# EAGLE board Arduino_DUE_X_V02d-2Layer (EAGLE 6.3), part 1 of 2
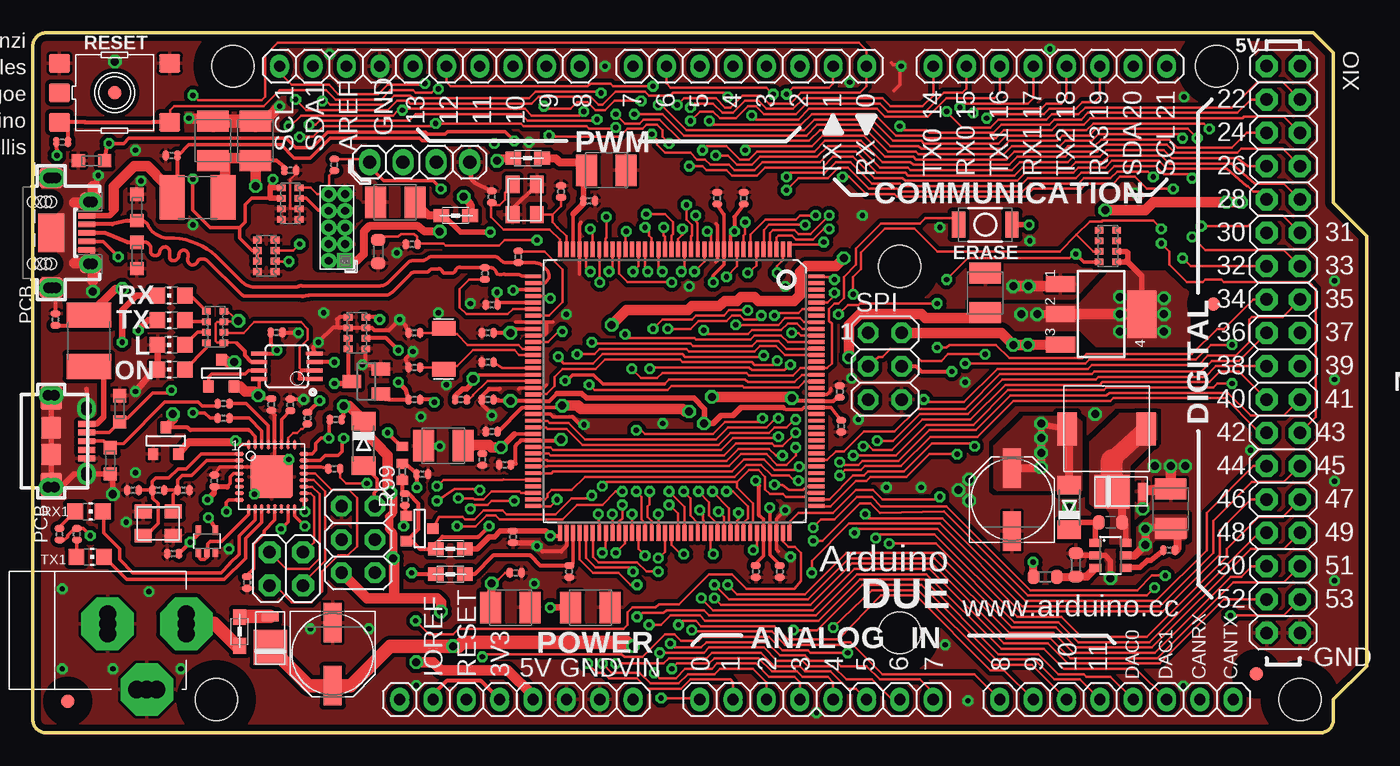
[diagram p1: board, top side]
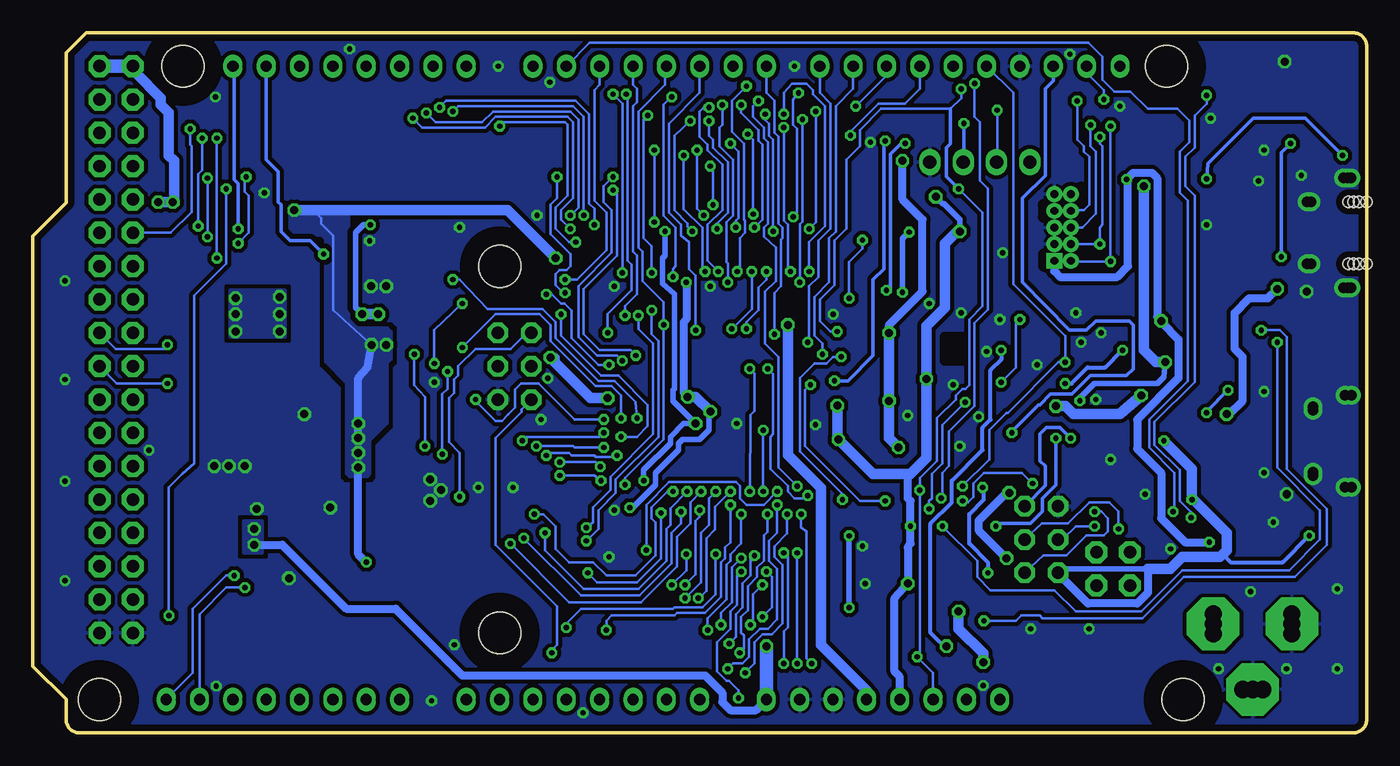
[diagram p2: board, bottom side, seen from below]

Size 101.6 x 53.34 mm. Coordinates in mm from the lower left corner, seen from the top.
Outline: 97.54,53.34 99.06,51.82 99.06,40.39 101.6,37.85 101.6,5.08 99.06,2.54 99.06,1 arc-90 98.06,0 1,0 arc-90 0,1 0,52.34 arc-90 1,53.34 97.54,53.34
Copper layers (1*16): Top 0.035mm / dielectric 1.6mm / Bottom 0.035mm
Design rules "default *": minimum track width 8mil, minimum drill 16mil, track to track 8mil, track to pad 8mil, pad to pad 8mil, via to via 8mil, smd to smd 6mil, copper to edge 20mil, drill to drill 12mil, minimum pad ring 12mil, minimum via ring 8mil, stop-mask expansion 2mil, vias tented up to drill 25mil, thermal gap 8mil
Net classes: 0 default: width 0.203 mm, drill 0.406 mm, clearance 0.203 mm; 1 USB: width 0.203 mm, drill 0.406 mm, clearance 0.203 mm; 2 gnd: width 0.203 mm, drill 0.406 mm, clearance 0.203 mm; 3 usbvcc: width 0.203 mm, drill 0.406 mm, clearance 0.203 mm; 4 USBpair: width 0.254 mm, drill 0.406 mm, clearance 0.61 mm
Holes 3.2 mm at 96.52,2.54 15.24,50.8 90.17,50.8 13.97,2.54 66.04,35.56 66.04,7.62
tRestrict: area 63.5,5.1 to 68.6,10.2; area 12.7,48.3 to 17.8,53.3; area 63.5,33 to 68.6,38.1; area 87.6,48.3 to 92.7,53.3; area 94,0 to 99.1,5.1; area 11.4,0 to 16.5,5.1; 5 lines
bRestrict: area 63.5,5.1 to 68.6,10.2; area 12.7,48.3 to 17.8,53.3; area 63.5,33 to 68.6,38.1; area 87.6,48.3 to 92.7,53.3; area 94,0 to 99.1,5.1; area 11.4,0 to 16.5,5.1; 5 lines

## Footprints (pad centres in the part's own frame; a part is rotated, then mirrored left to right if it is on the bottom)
1X08 = drill 0.85 pad 1.422 long: 1 -8.89,0; 2 -6.35,0; 3 -3.81,0; 4 -1.27,0; 5 1.27,0; 6 3.81,0; 7 6.35,0; 8 8.89,0
J0402 = smd 0.7 x 0.9: 1 -0.65,0; 2 0.65,0; 3 1.95,0
SMC_B = smd 1.6 x 2.4: + -1.5,0; - 1.5,0
C0402 = smd 0.508 x 0.762: 1 -0.445,0; 2 0.445,0
C0603-ROUND = smd 0.898 x 1.1: 1 -0.889,0; 2 0.889,0
MINIMELF = smd 1.4 x 1.8: A 1.7,0; C -1.7,0
DO220AAL = smd 2.667 x 2.54: P$1 -0.7,0 | smd 0.762 x 1.27: P$2 1.65,0
1X04 = drill 1.016 long: 1 -3.81,0; 2 -1.27,0; 3 1.27,0; 4 3.81,0
SMD_157SW = smd 1.016 x 1.981: 1 -2.032,0; 2 2.032,0
L1812 = smd 1.9 x 3.4: 1 -1.95,0; 2 1.95,0
FIDUCIA-MOUNT = smd 1.016 x 1.016: P$1 0,0
MSOP08 = smd 0.3 x 1.2: 1 -0.976,-2.113; 2 -0.326,-2.113; 3 0.324,-2.113; 4 0.974,-2.113; 5 0.974,2.112; 6 0.324,2.112; 7 -0.326,2.112; 8 -0.976,2.112
SOT23-6 = smd 0.6 x 0.9: 1 -0.95,-1.15; 2 0,-1.15; 3 0.95,-1.15; 4 0.95,1.15; 5 0,1.15; 6 -0.95,1.15
SOT223 = smd 1.219 x 2.235: 1 -2.311,-3.099; 2 0,-3.099; 3 2.311,-3.099 | smd 3.6 x 2.2: 4 0,3.099
MLF32 = smd 0.7 x 0.28: 1 -2.45,1.75; 2 -2.45,1.25; 3 -2.45,0.75; 4 -2.45,0.25; 5 -2.45,-0.25; 6 -2.45,-0.75; 7 -2.45,-1.25; 8 -2.45,-1.75; 17 2.45,-1.75; 18 2.45,-1.25; 19 2.45,-0.75; 20 2.45,-0.25; 21 2.45,0.25; 22 2.45,0.75; 23 2.45,1.25; 24 2.45,1.75 | smd 0.28 x 0.7: 9 -1.75,-2.45; 10 -1.25,-2.45; 11 -0.75,-2.45; 12 -0.25,-2.45; 13 0.25,-2.45; 14 0.75,-2.45; 15 1.25,-2.45; 16 1.75,-2.45; 25 1.75,2.45; 26 1.25,2.45; 27 0.75,2.45; 28 0.25,2.45; 29 -0.25,2.45; 30 -0.75,2.45; 31 -1.25,2.45; 32 -1.75,2.45 | smd 3.254 x 3.254: 33 0,0
SC70-5 = smd 0.4 x 0.7: 1 -0.65,-0.85; 2 0,-0.85; 3 0.65,-0.85; 4 0.65,0.85; 5 -0.65,0.85
2X03 = drill 0.95 pad 1.55 octagon: 1 -2.54,-1.27; 2 -2.54,1.27; 3 0,-1.27; 4 0,1.27; 5 2.54,-1.27; 6 2.54,1.27
CON2_USB_MICRO_B_AT = smd 0.406 x 1.346: P1 -1.321,2.692; P2 -0.66,2.692; P3 0,2.692; P4 0.66,2.692; P5 1.321,2.692 | drill 0.8 pad 1.27: P$1 -2.616,2.692 | drill 0.8 pad 1.245: P$2 -2.362,2.692; P$7 2.362,2.692; P$8 2.616,2.692 | drill 0.8 pad 1.143: P$3 -3.505,-0.254; P$4 -3.505,0.254; P$5 3.505,0.254; P$6 3.505,-0.254 | smd 1.778 x 1.651: S1 -3.302,0; S2 3.302,0 | smd 1.524 x 1.27: S3 -2.489,2.692; S4 2.489,2.692 | smd 1.626 x 1.524: S5 -1.016,0; S6 1.016,0
2X02 = drill 0.95 pad 1.676 octagon: 1 -1.27,-1.27; 2 -1.27,1.27; 3 1.27,-1.27; 4 1.27,1.27
R0402 = smd 0.508 x 0.762: 1 -0.445,0; 2 0.445,0
PINHEAD_2X05_127 = drill 0.6 pad 1.016 square: 1 -0.635,2.54 | drill 0.6 pad 1.016: 2 0.635,2.54; 3 -0.635,1.27; 4 0.635,1.27; 5 -0.635,0; 6 0.635,0; 7 -0.635,-1.27; 8 0.635,-1.27; 9 -0.635,-2.54; 10 0.635,-2.54
CHIP-LED0805 = smd 1.2 x 1.2: A 0,-1.05; C 0,1.05
0805 = smd 1.2 x 1: 1 -1.1,0; 2 1.1,0
SRR0604 = smd 1.5 x 2.5: P$1 3,0; P$2 -3,0
PANASONIC_D = smd 3 x 1.4: + 2.4,0; - -2.4,0
1X10 = drill 0.85 pad 1.422 long: 1 -11.43,0; 2 -8.89,0; 3 -6.35,0; 4 -3.81,0; 5 -1.27,0; 6 1.27,0; 7 3.81,0; 8 6.35,0; 9 8.89,0; 10 11.43,0
SOT23 = smd 1 x 1.4: 1 -0.95,-1.1; 2 0.95,-1.1; 3 0,1.1
R0603-ROUND = smd 0.898 x 1.1: 1 -0.889,0; 2 0.889,0
TS42 = smd 1.6 x 1.4: 1 -4.2,2.25; 2 4.2,2.25; 3 -4.2,-2.25; 4 4.2,-2.25; 5 -4.2,0
CAT16 = smd 0.5 x 0.65: 1 -1.2,-0.675; 2 -0.4,-0.675; 3 0.4,-0.675; 4 1.2,-0.675; 5 1.2,0.675; 6 0.4,0.675; 7 -0.4,0.675; 8 -1.2,0.675
CAY16 = smd 0.5 x 0.65: 1 -1.2,-0.675; 2 -0.4,-0.675; 3 0.4,-0.675; 4 1.2,-0.675; 5 1.2,0.675; 6 0.4,0.675; 7 -0.4,0.675; 8 -1.2,0.675
SOT-23 = smd 0.787 x 0.889: 1 0.025,-1.016; 2 -0.94,1.016; 3 0.991,1.016
LQFP144 = smd 0.3 x 1.2: 1 -8.75,-10.8; 2 -8.25,-10.8; 3 -7.75,-10.8; 4 -7.25,-10.8; 5 -6.75,-10.8; 6 -6.25,-10.8; 7 -5.75,-10.8; 8 -5.25,-10.8; 9 -4.75,-10.8; 10 -4.25,-10.8; 11 -3.75,-10.8; 12 -3.25,-10.8; 13 -2.75,-10.8; 14 -2.25,-10.8; 15 -1.75,-10.8; 16 -1.25,-10.8; 17 -0.75,-10.8; 18 -0.25,-10.8; 19 0.25,-10.8; 20 0.75,-10.8; 21 1.25,-10.8; 22 1.75,-10.8; 23 2.25,-10.8; 24 2.75,-10.8; 25 3.25,-10.8; 26 3.75,-10.8; 27 4.25,-10.8; 28 4.75,-10.8; 29 5.25,-10.8; 30 5.75,-10.8; 31 6.25,-10.8; 32 6.75,-10.8; 33 7.25,-10.8; 34 7.75,-10.8; 35 8.25,-10.8; 36 8.75,-10.8; 73 8.75,10.8; 74 8.25,10.8; 75 7.75,10.8; 76 7.25,10.8; 77 6.75,10.8; 78 6.25,10.8; 79 5.75,10.8; 80 5.25,10.8; 81 4.75,10.8; 82 4.25,10.8; 83 3.75,10.8; 84 3.25,10.8; 85 2.75,10.8; 86 2.25,10.8; 87 1.75,10.8; 88 1.25,10.8; 89 0.75,10.8; 90 0.25,10.8; 91 -0.25,10.8; 92 -0.75,10.8; 93 -1.25,10.8; 94 -1.75,10.8; 95 -2.25,10.8; 96 -2.75,10.8; 97 -3.25,10.8; 98 -3.75,10.8; 99 -4.25,10.8; 100 -4.75,10.8; 101 -5.25,10.8; 102 -5.75,10.8; 103 -6.25,10.8; 104 -6.75,10.8; 105 -7.25,10.8; 106 -7.75,10.8; 107 -8.25,10.8; 108 -8.75,10.8 | smd 1.2 x 0.3: 37 10.8,-8.75; 38 10.8,-8.25; 39 10.8,-7.75; 40 10.8,-7.25; 41 10.8,-6.75; 42 10.8,-6.25; 43 10.8,-5.75; 44 10.8,-5.25; 45 10.8,-4.75; 46 10.8,-4.25; 47 10.8,-3.75; 48 10.8,-3.25; 49 10.8,-2.75; 50 10.8,-2.25; 51 10.8,-1.75; 52 10.8,-1.25; 53 10.8,-0.75; 54 10.8,-0.25; 55 10.8,0.25; 56 10.8,0.75; 57 10.8,1.25; 58 10.8,1.75; 59 10.8,2.25; 60 10.8,2.75; 61 10.8,3.25; 62 10.8,3.75; 63 10.8,4.25; 64 10.8,4.75; 65 10.8,5.25; 66 10.8,5.75; 67 10.8,6.25; 68 10.8,6.75; 69 10.8,7.25; 70 10.8,7.75; 71 10.8,8.25; 72 10.8,8.75; 109 -10.8,8.75; 110 -10.8,8.25; 111 -10.8,7.75; 112 -10.8,7.25; 113 -10.8,6.75; 114 -10.8,6.25; 115 -10.8,5.75; 116 -10.8,5.25; 117 -10.8,4.75; 118 -10.8,4.25; 119 -10.8,3.75; 120 -10.8,3.25; 121 -10.8,2.75; 122 -10.8,2.25; 123 -10.8,1.75; 124 -10.8,1.25; 125 -10.8,0.75; 126 -10.8,0.25; 127 -10.8,-0.25; 128 -10.8,-0.75; 129 -10.8,-1.25; 130 -10.8,-1.75; 131 -10.8,-2.25; 132 -10.8,-2.75; 133 -10.8,-3.25; 134 -10.8,-3.75; 135 -10.8,-4.25; 136 -10.8,-4.75; 137 -10.8,-5.25; 138 -10.8,-5.75; 139 -10.8,-6.25; 140 -10.8,-6.75; 141 -10.8,-7.25; 142 -10.8,-7.75; 143 -10.8,-8.25; 144 -10.8,-8.75
MCR-AB1-S-RA-SMT = smd 0.4 x 1.35: 1 -1.3,2.7; 2 -0.65,2.7; 3 0,2.7; 4 0.65,2.7; 5 1.3,2.7 | drill 0.8: P$1 -4.175,0.356; P$3 -4.175,0.076; P$4 -4.175,-0.203; P$5 4.175,0.356; P$6 4.175,0.076; P$7 4.175,-0.203 | smd 2.9 x 2: P$2 0,0 | drill 0.8 pad 1.27: P$8 -2.35,3.15; P$9 -2.35,2.85; P$10 2.35,3.15; P$11 2.35,2.85 | smd 1.3 x 1.6: S1 -2.4,3; S2 2.4,3 | smd 1.5 x 1.8: S3 -4.175,0; S4 4.175,0 | hole 0.85: -2.375,0; 2.375,0; -2.375,-1.4; 2.375,-1.4; -2.375,-0.4; 2.375,-0.4; 2.375,-0.8; -2.375,-0.8
POWERSUPPLY_DC-21MM = drill 1.3 pad 4 octagon: 1 -5.08,-3.353; 2 -0.076,-6.35; 3 -0.076,-0.356 | drill 1.3: 4 -5.08,-4.115; 5 -5.08,-2.591; 6 -0.838,-0.356; 7 0.686,-0.356; 8 -0.838,-6.35; 9 0.686,-6.35
2X18 = drill 0.95 pad 1.676 octagon: 1 -21.59,-1.27; 2 -21.59,1.27; 3 -19.05,-1.27; 4 -19.05,1.27; 5 -16.51,-1.27; 6 -16.51,1.27; 7 -13.97,-1.27; 8 -13.97,1.27; 9 -11.43,-1.27; 10 -11.43,1.27; 11 -8.89,-1.27; 12 -8.89,1.27; 13 -6.35,-1.27; 14 -6.35,1.27; 15 -3.81,-1.27; 16 -3.81,1.27; 17 -1.27,-1.27; 18 -1.27,1.27; 19 1.27,-1.27; 20 1.27,1.27; 21 3.81,-1.27; 22 3.81,1.27; 23 6.35,-1.27; 24 6.35,1.27; 25 8.89,-1.27; 26 8.89,1.27; 27 11.43,-1.27; 28 11.43,1.27; 29 13.97,-1.27; 30 13.97,1.27; 31 16.51,-1.27; 32 16.51,1.27; 33 19.05,-1.27; 34 19.05,1.27; 35 21.59,-1.27; 36 21.59,1.27
CRYSTAL-3.2-2.5 = smd 1.3 x 1.05: 1 -1.15,-0.925; 2 1.15,-0.925; 3 1.15,0.925; 4 -1.15,0.925
RESONATOR_EPSON_FC_145 = smd 1.1 x 1.8: P$1 -1.55,0; P$2 1.55,0
CT/CN0603 = smd 1 x 1: 1 -1,0; 2 1,0

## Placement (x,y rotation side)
ADCH  8x1F-H8.5  [1X08]  82.55,2.54 0 top
ADCL  8x1F-H8.5  [1X08]  59.69,2.54 0 top
BR1  NM  [J0402]  28.14,21.18 270 top
C1  10u  [SMC_B]  36.37,9.55 0 top
C2  10u  [SMC_B]  27.61,40.44 180 top
C3  10u  [SMC_B]  42.47,9.55 0 top
C4  100n  [C0402]  35.97,20.42 0 top
C5  100n  [C0402]  52.12,40.74 270 top
C6  100n  [C0402]  34.95,22.96 0 top
C7  100n  [C0402]  56.9,12.29 90 top
C8  100n  [C0402]  61.47,26.01 270 top
C9  100n  [C0402]  34.95,32.61 0 top
C10  100n  [C0402]  36.58,14.94 90 top
C11  10u  [SMC_B]  31.27,21.87 180 top
C12  100n  [C0402]  34.24,20.83 90 top
C13  100n  [C0402]  54.15,40.74 270 top
C14  100n  [C0402]  34.65,30.48 0 top
C15  100n  [C0402]  34.65,25.4 0 top
C16  100n  [C0402]  55.07,12.29 90 top
C17  100n  [C0402]  61.57,23.37 90 top
C18  100n  [C0402]  36.78,12.19 180 top
C19  100n  [C0402]  40.84,12.29 90 top
C20  10n  [C0402]  2.24,45.01 180 top
C21  22p  [C0402]  40.23,41.25 90 top
C22  22p  [C0402]  34.95,40.84 90 top
C23  22pF_NM  [C0402]  29.06,27.84 180 top
C24  22pF_NM  [C0402]  29.06,30.48 180 top
C25  22p  [C0402]  28.85,37.24 180 top
C26  10n  [C0402]  10.57,43.99 180 top
C27  10u  [SMC_B]  16.97,45.11 90 top
C28  100n  [C0402]  1.73,31.5 90 top
C29  10u  [SMC_B]  72.54,33.53 90 top
C30  100n  [C0402]  18.16,25.02 90 top
C31  100n  [C0402]  18.57,30.51 180 top
C32  100n  [C0402]  42.37,40.54 180 top
C33  10u  [SMC_B]  43.69,42.88 0 top
C34  100n  [C0402]  29.67,19.71 180 top
C35  10u  [SMC_B]  13.72,45.11 90 top
C36  100n  [C0402]  13.82,19.2 90 top
C37  100n  [C0402]  10.69,13.65 180 top
C38  1u  [C0402]  19.61,24.99 90 top
C39  22p  [C0402]  7.62,18.49 180 top
C40  22p  [C0402]  11.48,18.49 0 top
C41  10u  [SMC_B]  86.66,17.07 90 top
C42  10n  [C0603-ROUND]  82.09,16.05 0 top
COMMUNICATION  8x1F-H8.5  [1X08]  77.47,50.8 0 top
D2  CD1206-S01575  [MINIMELF]  25.2,22.05 270 top
D3  CD1206-S01575  [MINIMELF]  78.94,17.17 90 top
D4  SS1P3L  [DO220AAL]  82.91,18.39 0 top
D5  SS1P3L  [DO220AAL]  18.08,7.21 90 top
DEBUG  STRIP 4x1V M  [1X04]  29.46,43.48 180 top
ERASE  [SMD_157SW]  72.54,38.71 180 top
F1  MF-MSMF050-2 500mA  [L1812]  12.55,40.79 180 top
F2  MF-MSMF050-2 500mA  [L1812]  4.27,29.87 270 top
FID1  FIDUCIALMOUNT  [FIDUCIA-MOUNT]  89.92,32.68 0 top
FID2  FIDUCIALMOUNT  [FIDUCIA-MOUNT]  93.19,4.5 0 top
FID3  FIDUCIALMOUNT  [FIDUCIA-MOUNT]  6.22,48.77 0 top
FID4  FIDUCIALMOUNT  [FIDUCIA-MOUNT]  2.67,2.41 0 top
IC1  LMV358IDGKR  [MSOP08]  19.35,27.94 90 top
IC2  LM2734Y  [SOT23-6]  82.09,13.51 270 top
IC4  NCP1117ST33T3G -3V3  [SOT223]  81.38,31.9 270 top
IC6  ATMEGA16U2-MU  [MLF32]  18.19,19.51 0 top
IC10  74LVC1G125DCK  [SC70-5]  13.26,14.6 0 top
ICSP1  3x2M  [2X03]  24.79,14.73 90 top
J3  USB-MICRO B  [CON2_USB_MICRO_B_AT]  1.4,22.23 270 top
JP5  2x2M - NM  [2X02]  19.31,12.5 180 top
JR1  0R  [R0402]  28.14,19.91 90 top
JTAG  [PINHEAD_2X05_127]  23.16,38.51 180 top
L  YELLOW  [CHIP-LED0805]  10.54,29.57 90 top
L1  MH2029-300Y  [0805]  31.8,14.02 0 top
L2  MH2029-300Y  [0805]  32.21,39.42 180 top
L3  MH2029-300Y  [0805]  31.8,12.09 0 top
L4  10u SRR0604-100ML  [SRR0604]  81.79,23.16 0 top
L5  MH2029-300Y  [0805]  37.69,43.79 0 top
L6  MH2029-300Y  [0805]  15.75,7.72 270 top
ON  GREEN  [CHIP-LED0805]  10.54,27.69 90 top
PC1  47u  [PANASONIC_D]  22.83,5.99 270 top
PC2  47u  [PANASONIC_D]  74.57,17.78 90 top
POWER  8x1F-H8.5  [1X08]  36.83,2.54 0 top
PWMH  10x1F-H8.5  [1X10]  30.23,50.8 180 top
PWML  8x1F-H8.5  [1X08]  54.61,50.8 180 top
Q2  BC847BSMD  [SOT23]  25.4,26.77 90 top
R1  0R  [R0402]  22.96,43.28 90 top
R2  10K  [R0402]  19.61,42.88 180 top
R3  1K  [R0402]  29.06,25.4 180 top
R4  100K  [R0402]  32.61,25.4 180 top
R5  39R 1%  [R0402]  36.98,36.27 90 top
R6  39R 1%  [R0402]  34.44,35 270 top
R7  6k8 1%  [R0603-ROUND]  26.31,36.68 90 top
R8  0R_NM  [R0402]  34.65,28.24 0 top
R9  1M_NM  [R0402]  9.55,18.49 0 top
R10  10k  [R0402]  86.56,13.92 180 top
R11  10K  [R0603-ROUND]  79.45,12.8 90 top
R12  52K3  [R0603-ROUND]  77.11,11.89 0 top
R13  10K  [R0402]  23.06,23.88 0 top
R14  1K  [R0402]  3.35,15.14 270 top
R15  1K  [R0402]  2.03,15.14 90 top
R18  10K  [R0402]  16.31,11.46 270 top
R19  22R  [R0402]  14.53,23.98 180 top
R20  22R  [R0402]  14.53,25.1 180 top
R21  1K  [R0402]  20.93,23.98 90 top
R23  1K  [R0402]  22.96,20.12 0 top
R99  10K  [R0402]  28.35,17.78 90 top
RESET  TS42  [TS42]  6.22,48.77 0 top
RN1  100K  [CAT16]  19.61,40.34 90 top
RN2  100K  [CAT16]  17.78,36.35 270 top
RN3  1k  [CAY16]  13.89,30.94 270 top
RN4  100K  [CAT16]  24.69,30.48 270 top
RN5  1K5  [CAT16]  81.89,37.08 90 top
RX  YELLOW  [CHIP-LED0805]  10.54,33.32 90 top
RX1  YELLOW  [CHIP-LED0805]  4.27,16.87 270 top
SPI  3x2M  [2X03]  64.9,27.94 270 top
T1  FDN340P  [SOT-23]  14.38,27.41 180 top
T2  FDN340P  [SOT-23]  10.16,22.25 180 top
T3  FDN340P  [SOT-23]  29.46,15.54 90 top
TX  YELLOW  [CHIP-LED0805]  10.54,31.45 90 top
TX1  YELLOW  [CHIP-LED0805]  4.37,13.41 270 top
U1  ATSAM3X8EA-AU  [LQFP144]  48.9,26.04 180 top
USB1  MICRO-USB-AB1  [MCR-AB1-S-RA-SMT]  1.4,38.1 270 top
X2  POWERSUPPLY_DC21MMX  [POWERSUPPLY_DC-21MM]  5.33,8.38 90 top
XIO  18x2F-H8.5  [2X18]  95.25,29.21 270 top
Y1  12MHz KX-7 20pF  [CRYSTAL-3.2-2.5]  37.47,40.64 270 top
Y2  32.768Khz  [RESONATOR_EPSON_FC_145]  31.29,29.26 90 top
Y4  16MHz KX-7 20pF  [CRYSTAL-3.2-2.5]  9.55,15.95 0 top
Z1  CG0603MLC-05E  [CT/CN0603]  7.92,36.37 270 top
Z2  CG0603MLC-05E  [CT/CN0603]  7.92,40.03 90 top
Z3  CG0603MLC-05E  [CT/CN0603]  6.6,24.69 270 top
Z4  CG0603MLC-05E  [CT/CN0603]  5.89,20.73 90 top
Z5  CG0603MLC-05E  [CT/CN0603]  4.47,43.59 0 top

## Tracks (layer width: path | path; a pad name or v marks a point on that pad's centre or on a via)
8PB4
  Top 0.203: IC6.18 21.16,18.26 21.44,17.98 21.44,14.53 JP5.1
8PB5
  Top 0.203: IC6.19 21.27,18.76 21.84,18.19 21.84,13.31 21.03,12.5 19.31,12.5 JP5.3
8PB6
  Top 0.203: IC6.20 21.38,19.26 22.25,18.39 22.25,13.11 20.58,11.43 JP5.2
8PB7
  Top 0.203: IC6.21 21.49,19.76 22.76,18.49 24.08,18.49 24.69,17.88 24.69,14.22 23.98,13.51 23.27,13.51 22.05,12.29 22.05,10.77 21.23,9.96 19.71,9.96 18.44,11.23 JP5.4
16U2-TX
  Top 0.254: IC6.9 16.44,16.64 14.4,14.6 13.5,14.6 13.3,14.4 13.3,13.79 IC10.2 13.26,13.37 13.11,13.21 12.8,13.21 12.61,13.4 IC10.1
+3V3  (via drill 0.41, 0.61)
  Top 0.203: C1.+ 34.95,9.55 | 38,24.79 U1.57 38.19,24.78 | 52.64,36.88 U1.11 | L2.1 33.36,39.45 33.33,39.62 | C18.2 35.97,12.19 35.46,11.68 v34.95,11.38 | 17.09,36.73 RN2.2 | 61.57,25.4 C8.2 | RN3.8 14.8,32.14 v15.65,31.39 15.59,31.34 RN3.7 14.52,31.29 14.02,31.29 13.92,31.19 13.92,29.87 14.05,29.74 RN3.5 15.51,29.74 15.54,29.67
  Top 0.254: 17.09,36.73 17.07,36.73 17.07,36.12 17.04,35.95 RN2.3 | C37.1 11.13,13.67 | RN2.2 16.69,36.75 15.75,37.69 15.75,38.51 | 15.75,38.51 13.51,38.51 12.19,39.83 v12.19,42.22 | 18.09,40.73 16.66,40.73 16.15,40.23 16.15,38.91 15.75,38.51 | RN5.2 82.8,36.68
  Top 0.279: 37.27,24.78 38,24.79 | U1.52 34.02,27.29 33.71,27.08 | v40.32,24.93 40.13,24.79 40.12,24.78 38.19,24.78 | v51.82,34.34 51.82,34.85 52.64,35.67 52.64,36.8 52.65,36.8 U1.11 | 52.64,36.88 52.64,39.5 | v56.13,17.17 56.15,17.23 U1.105 56.15,13.55 56.9,12.8 C7.2
  Top 0.305: 52.64,39.5 C5.2 | v57.81,25.5 58.03,25.29 U1.125 60.97,25.29 61.25,25.57 C8.2 | C4.2 36.78,20.52 36.78,21.89 37.17,22.29 U1.62 40.17,22.29 v40.23,22.35 | C20.2 v1.83,43.99 | JR1.1 BR1.3 28.14,18.43 R99.2 28.38,18.19 28.65,18.19 29.36,17.48 29.36,15.52 T3.2 28.68,14.81 29.46,14.02 L1.1 30.7,14.45 31.19,14.94 33.93,14.94 v34.75,15.75 | 11.13,13.67 v11.99,14.53 12.61,15.15 IC10.5 | IC1.6 16.64,28.26 16.15,28.75 16.15,29.06 15.54,29.67 | POWER.4 34.14,3.96 31.5,3.96 30.48,2.95 POWER.2 | C6.2 35.46,22.96 37.27,24.78
  Top 0.406: 33.71,27.08 v33.53,26.98 33.53,26.72 33.02,26.21 32.72,26.21 32.17,25.67 R4.2 | ERASE.1 v75.89,38.71 | 30.64,14.08 L1.1 | RN5.1 83.23,35.88 | 83.23,35.88 83.41,36.07 83.41,36.58 83.31,36.68 82.8,36.68 RN5.2 | 83.23,35.88 83.39,35.88 84.48,34.8 IC4.4 | RN1.6 18.09,40.73 18.09,41.55 | 18.09,41.55 18.32,41.55 RN1.5 | 18.09,41.55 v18.29,42.16 | RN5.2
  Top 0.61: v32.82,40.84 33.33,40.23 33.33,39.62 | v76.5,31.9 IC4.2 | v30.99,38.2 29.87,38.2 29.36,38.61 25.6,38.61 25.2,38.2 25.2,36.47 24.69,35.97 JTAG.1 | 34.95,9.55 v34.95,11.38
  Top 0.813: IC4.2 IC4.4 | v62.18,28.6 62.18,31.09 62.99,31.9 67.67,31.9 67.97,31.6 72.21,31.6 C29.+ 72.67,31.9 | v51.71,25.6 57.71,25.6 v57.81,25.5 | v40.32,24.93 41.52,24.93 41.76,24.69 49.48,24.69 49.68,24.49 v49.99,24.49
  Bottom 0.254: v12.19,42.22 12.09,43.38 8.64,46.84 4.67,46.84 v1.83,43.99
  Bottom 0.406: v75.89,38.71 76.4,38.71 77.01,38.1 77.01,32.41 v76.5,31.9 | 18.19,42.06 v18.29,42.16 | v49.99,24.49 50.09,24.38 50.09,23.06 50.8,22.35 52.12,22.35 52.43,22.05 52.43,21.54 54.15,19.81 54.15,18.9 55.88,17.17 v56.13,17.17 | v40.23,22.35 40.32,22.47 | v30.99,38.2 30.99,39.12 32.21,40.34 32.31,40.34 v32.82,40.84 | v15.65,31.39 15.65,31.29
  Bottom 0.61: JTAG.1 23.8,35.18 23.37,34.75 19,34.75 18.19,35.56 18.19,42.06 | v18.29,42.16 17.78,42.67 16.36,42.67 15.95,42.27 15.95,31.7 v15.65,31.39 | v51.82,34.34 51.82,31.5 52.02,31.29 52.02,25.91 v51.71,25.6 | POWER.4 35.56,4.27 35.97,4.67 35.97,10.26 v34.95,11.38 34.95,14.12 34.75,14.43 v34.75,15.75 34.75,17.68 34.95,17.88 34.95,19.51 34.75,19.71 | 15.65,31.29 14.33,29.97 14.33,27.03 17.48,23.88 17.48,21.64 15.65,19.81 15.65,16.36 13.82,14.53 v11.99,14.53
  Bottom 0.813: v75.29,31.9 v76.5,31.9 | v51.71,25.6 51.1,25.6 v49.99,24.49 | 40.32,22.47 v40.32,24.93 | v40.23,22.35 37.59,19.71 34.75,19.71 33.53,20.93 v33.53,26.98 33.53,30.99 32.11,32.41 32.11,37.29 31.19,38.2 v30.99,38.2 | v62.18,28.6 61.87,28.55 61.87,28.25 59.13,25.5 v57.81,25.5
  other vias: 82.8,33.22 82.8,31.9 86.16,33.12 86.16,31.9 82.8,30.58 86.16,30.58
  pour Top (isolate 0.406, no thermals): 71.42,31.19 71.42,32.61 79.65,32.61 81.99,35.15 86.46,35.15 88.09,33.53 88.09,29.67 87.48,29.16 81.58,29.06 81.38,29.06 79.76,30.68 74.47,30.68 73.96,31.19
  pour Bottom: 82.4,33.73 86.56,33.73 86.56,30.18 82.4,30.18 82.4,33.63
+5V  (via drill 0.41, 0.61)
  Top 0.254: IC6.4 15.29,19.76 15.04,19.51 15.04,19 14.79,18.76 | IC6.32 15.74,21.96 v15.44,22.25 | v4.37,15.04 3.82,15.58 R14.1 3.19,15.58 2.64,15.04 2.64,14.94 2.4,14.69 R15.1 | IC1.8 17.24,25.78 v17.17,25.7
  Top 0.305: C30.2 17.41,25.46 v17.17,25.7 | R13.2 23.67,24.14 v23.67,24.89
  Top 0.406: 25.3,23.98 25.27,23.98 D2.C | 14.79,18.76 C36.1 13.83,18.3 v13.31,17.78 | 15.34,22.15 v15.44,22.25
  Top 0.508: L4.P$2 77.01,23.47 76.81,23.27 v76.81,22.45
  Top 0.61: PC2.+ 76.77,20.18 v76.81,20.22 v76.81,21.34 v76.81,22.45 | R12.1 v76.2,13.01 | D3.A 78.94,23.31 L4.P$2 | T2.2 11.89,22.15 15.34,22.15 | 27.03,18.49 27.43,18.09 27.43,16.76 27.13,16.46 27.13,15.54 27.43,15.24 v27.43,13.31
  Top 0.813: v29.21,5.38 30.48,5.38 31.09,4.78 36.17,4.78 38.1,2.85 POWER.5 | v81.69,39.83 84.73,39.83 85.34,40.44 v90.93,40.44 v92.05,40.44 | v44.09,31.09 45.21,32.21 49.89,32.21 50.19,32.51 52.27,32.51 52.73,32.92 53.65,32.92 53.95,33.22 54.97,33.22 55.27,32.92 57.96,32.92 58.42,33.38 58.42,35.1 58.88,35.56 61.16,35.56 v61.77,36.17 | v75.79,29.57 78.05,29.59 IC4.3 76.12,29.57 v74.68,29.57 73.76,30.48 SPI.2 | 23.71,24.95 v23.67,24.89 24.08,24.89 24.99,23.98 25.27,23.98 | T1.2 15.77,26.39 16.15,26.01 16.87,26.01 v17.17,25.7 | v31.09,9.25 31.09,9.96 30.79,10.26 27.53,10.26 | ICSP1.2 25.45,10.26 27.53,10.26 | D2.C 25.4,22.86 27.03,21.13 27.03,18.49 | 27.53,10.26 27.53,12.9 27.43,13.11 v27.43,13.31
  Bottom 0.203: 80.16,39.83 80.16,39.73 79.65,39.22 79.65,38.81 78.74,37.9 78.74,32.21 v75.79,29.57
  Bottom 0.305: v4.37,15.04 6.4,13.01 10.36,13.01 10.97,13.61
  Bottom 0.406: 13.21,17.78 v13.31,17.78 | ICSP1.2 23.16,12.5 16.66,12.5
  Bottom 0.61: v76.81,22.45 76.81,27.03 76.1,27.84 v75.79,29.57 | v76.2,13.01 76.81,13.61 v76.81,20.22 | 11.18,13.41 10.97,13.61 | 16.66,12.5 16.66,10.67 17.48,9.86 21.23,9.86 23.57,12.19 | v27.23,18.29 27.43,18.29 29.57,16.15 29.57,15.44 v27.43,13.31
  Bottom 0.813: XIO.1 93.78,50.29 91.85,48.36 91.85,47.85 91.24,47.24 91.24,43.99 90.83,43.59 90.83,40.64 91.03,40.44 | v44.09,31.09 44.09,21.18 41.55,18.64 41.55,6.71 38.1,3.25 POWER.5 | v61.77,36.17 65.43,39.83 80.16,39.83 v81.69,39.83 | v90.93,40.44 91.03,40.44 | 91.03,40.44 v92.05,40.44 | v13.31,17.78 13.31,20.12 v15.44,22.25 | v23.67,24.89 22.96,24.89 22.35,24.28 18.8,24.28 v17.17,25.7 | v29.21,5.38 29.21,6.04 31.09,7.92 v31.09,9.25 | 16.66,12.5 14.94,12.5 14.02,13.41 11.18,13.41 | 10.97,13.61 10.67,13.92 10.67,15.23 13.21,17.78
  Bottom 1.016: XIO.1 XIO.2
  other vias: 76.81,23.57
  pour Top (isolate 0.406, no thermals): 79.45,24.08 75.49,24.08 73.25,21.84 73.25,18.69 73.46,18.49 79.86,18.49 79.86,23.67
  pour Bottom (isolate 0.406): 74.27,30.58 74.27,28.45 74.57,28.14 74.57,23.57 75.9,22.25 75.9,19.71 76.1,19.51 77.52,19.51 77.72,19.71 77.72,26.62 79.35,28.24 79.35,37.59 79.65,37.9 81.58,37.9 82.3,38.61 82.3,40.13 77.52,40.13 77.52,31.6 76.81,30.89 74.57,30.89
AD0  (via drill 0.41)
  Top 0.203: v47.65,12.29 46.74,12.29 46.02,13.01 43.08,13.01 42.67,13.41 42.67,15.04 U1.78 | ADCL.1 50.8,2.64 v47.85,2.64
  Bottom 0.203: v47.65,12.29 47.95,11.99 47.95,9.75 48.46,9.25 48.46,7.92 49.48,6.91 49.48,4.67 48.77,3.96 48.56,3.96 47.85,3.25 v47.85,2.64
AD1  (via drill 0.41)
  Top 0.203: U1.79 43.18,15.23 43.18,16.05 43.08,16.15 v43.08,16.66 | v42.27,5.28 42.98,4.57 43.48,4.57 43.89,4.17 46.02,4.17 46.84,3.35 49.38,3.35 50.09,4.06 53.14,4.06 53.34,3.86 ADCL.2
  Bottom 0.203: v43.08,16.66 43.08,15.65 42.67,15.34 42.67,5.69 v42.27,5.28
AD2  (via drill 0.41)
  Top 0.203: v43.38,13.72 43.64,13.92 U1.80 | ADCL.3 55.88,3.86 54.86,4.88 52.32,4.88 51.92,4.47 49.89,4.47 49.17,3.76 47.04,3.76 46.23,4.57 44.09,4.57 v43.38,5.28
  Bottom 0.203: v43.38,5.28 v43.38,13.72
AD3  (via drill 0.41)
  Top 0.203: U1.81 44.15,16.61 v44.15,16.66 | ADCL.4 58.42,3.86 58.01,4.27 56.08,4.27 55.07,5.28 52.12,5.28 51.71,4.88 49.68,4.88 48.97,4.17 47.75,4.17 v47.35,4.57
  Bottom 0.203: v44.15,16.66 44.15,15.19 45.11,14.22 45.11,13.41 44.5,12.8 44.5,8.33 45.31,7.52 46.02,7.52 46.63,6.91 46.63,5.28 v47.35,4.57
AD4  (via drill 0.41)
  Top 0.203: U1.82 44.65,16.09 44.91,16.36 v44.91,17.37 | 60.96,2.44 ADCL.5 60.96,3.86 60.55,4.27 58.62,4.27 58.22,4.67 56.29,4.67 55.27,5.69 51.92,5.69 51.51,5.28 49.07,5.28 v48.67,4.88
  Bottom 0.203: v44.91,17.37 44.91,15.24 45.52,14.63 45.52,13.11 44.91,12.5 44.91,8.64 45.62,7.92 46.23,7.92 47.04,7.11 47.04,5.79 47.55,5.28 48.26,5.28 v48.67,4.88
AD5  (via drill 0.41)
  Top 0.203: v44.4,13.72 45.11,14.43 45.11,15.04 U1.83 | v44.4,5.28 48.06,5.28 48.46,5.69 51.31,5.69 51.71,6.1 55.47,6.1 56.49,5.08 58.42,5.08 58.83,4.67 60.76,4.67 62.08,3.35 62.69,3.35 ADCL.6
  Bottom 0.203: v44.4,13.72 44.09,13.41 44.09,8.03 44.4,7.72 v44.4,5.28
AD6  (via drill 0.41)
  Top 0.203: U1.84 45.65,16.59 v45.64,16.66 | v47.75,6.1 51.1,6.1 51.51,6.5 55.68,6.5 56.69,5.49 58.62,5.49 59.03,5.08 60.96,5.08 61.98,4.06 63.91,4.06 65.43,2.54 ADCL.7
  Bottom 0.203: v47.75,6.1 47.45,6.4 47.45,7.42 47.65,7.62 47.65,8.84 47.14,9.35 47.14,11.18 46.43,11.89 46.43,12.6 45.92,13.11 45.92,15.04 45.64,15.32 v45.64,16.66
AD7  (via drill 0.41)
  Top 0.203: v46.63,13.51 46.58,13.56 46.13,14.02 46.13,15.04 U1.85 | ADCL.8 68.58,3.05 67.56,4.06 64.52,4.06 63.5,5.08 61.57,5.08 61.16,5.49 59.23,5.49 58.83,5.89 56.9,5.89 55.88,6.91 51.31,6.91 50.9,6.5 48.87,6.5 v48.56,6.81
  Bottom 0.203: v46.63,13.51 46.94,13.21 46.94,11.99 47.55,11.38 47.55,9.55 48.06,9.04 48.06,7.32 v48.56,6.81
AD8  (via drill 0.41)
  Top 0.203: U1.88 47.65,16.55 v47.65,16.66 | v50.19,7.82 50.29,7.72 56.29,7.72 57.3,6.71 61.57,6.71 61.77,6.91 62.28,6.91 64.72,4.47 71.73,4.47 ADCH.1
  Bottom 0.203: v47.65,16.66 47.65,14.43 48.46,13.61 48.46,13.11 48.77,12.8 48.77,10.16 50.19,8.74 v50.19,7.82
AD9  (via drill 0.41)
  Top 0.203: v49.17,8.23 49.48,8.53 50.49,8.53 50.9,8.13 56.49,8.13 57.51,7.11 61.37,7.11 64.62,10.46 67.26,10.46 72.95,4.78 73.97,4.78 ADCH.2 | U1.89 48.16,15.04 48.16,13.85 48.14,13.8 47.73,13.39 | 47.63,13.31 47.73,13.39 | 47.73,13.39 v47.65,13.31
  Bottom 0.203: v49.17,8.23 49.17,9.14 48.36,9.96 48.36,12.6 v47.65,13.31
AD10  (via drill 0.41)
  Top 0.203: v49.58,13.61 49.38,13.61 48.67,14.33 48.67,15.24 U1.90 | v60.96,8.03 63.91,10.87 67.46,10.87 73.15,5.18 76.1,5.18 ADCH.3
  Bottom 0.203: v49.58,13.61 49.58,10.57 50.6,9.55 52.73,9.55 52.83,9.45 59.84,9.45 60.96,8.33 v60.96,8.03
AD11(TXD3)  (via drill 0.41)
  Top 0.203: v57.91,7.82 59.74,7.82 63.2,11.28 67.67,11.28 73.36,5.59 76.3,5.59 77.83,4.06 79.76,4.06 ADCH.4 | U1.91 49.12,15.29 49.12,16.71 v48.46,17.37
  Bottom 0.203: v48.46,17.37 48.46,14.53 48.87,14.12 48.87,13.31 49.17,13.01 49.17,10.36 50.39,9.14 52.53,9.14 52.73,8.94 57.51,8.94 57.91,8.53 v57.91,7.82
AD14(RXD3)  (via drill 0.41)
  Top 0.203: U1.92 49.65,17.21 v48.46,18.39 | v50.9,10.26 51.82,9.35 59.44,9.35 62.59,12.5 68.28,12.5 73.97,6.81 77.32,6.81 78.84,5.28 85.85,5.28 90.73,10.16 XIO.33
  Bottom 0.203: v48.46,18.39 49.63,17.22 49.63,15.49 50.29,14.83 50.29,10.82 v50.9,10.26
AREF  (via drill 0.41)
  Top 0.305: BR1.1 27.94,21.95 v27.03,22.86
  Bottom 0.254: PWMH.8 23.88,49.68 24.49,49.07 24.49,42.47 26.21,40.74 26.21,34.34 22.66,30.68 21.34,30.68 20.62,31.39 18.09,31.39 17.78,31.09 17.78,27.74 18.29,27.23 21.03,27.23 22.45,25.81 24.08,25.81 24.89,24.99 24.99,24.99 26.82,23.16 v27.03,22.86
AVREF
  Top 0.203: 41.15,12.9 41.05,12.8 C19.2
  Top 0.279: U1.75 41.15,12.9
  Top 0.305: C19.2 38.67,12.74 37.9,13.51 35.05,13.51 33.63,12.09 L3.2
AVREFL  (via drill 0.41)
  Top 0.305: L3.1 28.96,12.09 v28.85,12.19 | v29.26,18.69 29.22,18.55 C34.2 28.4,20.53 BR1.2 JR1.2
  Bottom 0.305: v29.26,18.69 29.16,18.29 29.16,17.78 30.28,16.66 30.28,14.43 28.85,13.01 v28.85,12.19
BD+
  Top 0.254: J3.P3 4.12,22.25 5.38,22.25 5.89,21.74 Z4.2 5.99,22.03 6.91,22.05 10.06,25.2 12.6,25.2 12.9,24.89 13.88,24.89 R20.2
BD-  (via drill 0.41)
  Top 0.254: J3.P2 5.8,22.89 Z3.2 6.52,23.99 6.53,23.98 7.21,23.98 9.14,25.91 10.36,25.91 v10.57,26.11 | R19.2 13.51,23.98 13.11,24.38 v12.19,24.38
  Bottom 0.254: v10.57,26.11 12.19,24.49 v12.19,24.38
BOOST
  Top 0.406: IC2.1 80.94,15.89 C42.1 79.76,16.05 79.48,15.78 D3.C
CANRX0  (via drill 0.41)
  Top 0.203: v45.72,35.15 46.13,35.56 46.13,36.78 U1.24 | v85.45,11.07 84.84,10.46 75.79,10.46 69.39,16.87 64.52,16.76 63.8,17.48 62.99,17.48 60.15,14.63 v59.44,14.63 | v47.24,30.79 47.95,31.5 50.19,31.5 50.49,31.8 52.63,31.8 53.03,32.21 v54.46,32.21
  Bottom 0.203: v85.45,11.07 86.87,11.07 88.9,9.04 ADCH.7 | v54.46,32.21 54.46,30.38 53.95,29.87 53.95,22.55 57.2,19.3 57.2,18.29 58.52,16.97 58.52,15.54 v59.44,14.63 | v47.24,30.79 47.24,31.29 46.33,32.21 46.33,33.93 45.72,34.54 v45.72,35.15
CANTX0  (via drill 0.41)
  Top 0.203: U1.23 46.63,36.84 46.63,35.36 v46.84,35.15 | v48.36,30.79 50.09,30.79 50.7,31.39 52.83,31.39 53.24,31.8 53.85,31.8 54.15,31.5 55.17,31.5 v55.47,31.8 | v59.44,15.65 60.05,16.26 61.06,16.26 62.79,17.98 63.91,17.98 64.62,17.27 69.6,17.27 76,10.87 84.12,10.87 85.24,11.99 v86.26,11.99
  Bottom 0.203: v46.84,35.15 46.84,32.31 v48.36,30.79 | v55.47,31.8 55.47,30.79 54.36,29.67 54.36,22.76 57.61,19.51 57.61,18.49 58.93,17.17 58.93,16.05 v59.44,15.65 | v86.26,11.99 86.87,11.99 89.41,9.45 89.41,4.57 ADCH.8
CANTX1/IO  (via drill 0.41)
  Top 0.203: U1.140 60.52,32.78 61.06,33.33 v61.06,33.53 | v61.67,42.37 62.18,42.37 63.5,41.05 65.63,41.05 65.84,40.84 75.59,40.84 76.2,41.45 79.86,41.45 80.26,41.86 82.3,41.86 82.8,42.37 83.92,42.37 84.84,41.45 v86.87,41.45 | v91.24,8.94 95.3,8.94 XIO.34
  Bottom 0.203: v91.24,8.94 91.24,18.69 90.22,19.71 89.31,20.52 89.31,33.33 86.87,35.76 v86.87,41.45 | v61.67,42.37 61.67,40.74 62.18,40.23 62.18,38 60.66,36.47 60.66,35.56 60.96,35.26 61.47,35.26 61.77,34.95 61.77,34.14 61.16,33.53 v61.06,33.53
CMP  (via drill 0.41)
  Top 0.203: 17.07,28.91 IC1.5 | 24.18,26.62 Q2.3
  Top 0.305: 17.07,28.91 18.34,28.91 v18.59,29.16 18.12,29.63 C31.2 | 24.74,26.62 24.03,26.62 RN4.4 RN4.3
  Top 0.406: v22.96,26.62 24.03,26.62 24.18,26.62
  Bottom 0.305: v22.96,26.62 22.48,26.62 21.26,27.84 19.91,27.84 v18.59,29.16
D+
  Top 0.254: 37.3,34.8 37.95,34.8 U1.37 | 37.3,34.8 arc-45 37.28,34.81 | 7.92,37.39 8.53,37.39 arc-90 8.99,36.87 arc90 9.19,36.37 9.2,36.37 arc90 9.65,36.58 arc-90 10.11,37.03 arc-90 10.41,36.58 10.41,36.32 arc90 10.67,35.97 arc90 11.12,36.42 arc-90 11.53,36.78 arc-90 11.84,36.27 arc90 12.04,35.66 arc90 12.6,36.02 arc-67 13.27,36 15.81,33.46 arc45 16.22,33.27 20.46,33.27 arc45 20.76,33.31 20.97,33.32 arc-45 21.07,33.35 26.89,33.35 arc45 27.44,33.64 28.77,34.97 arc-45 29.07,35.1 29.95,35.1 arc45 30.13,35.16 arc-45 30.46,35.36 30.89,35.36 arc-90 31.19,35.15 arc90 31.39,35.05 31.8,35.05 arc90 32.21,35.26 arc-90 32.61,35.46 34.63,35.46 | 37.3,34.8 arc-45 37.28,34.81 | 34.39,35.46 R6.1 34.63,35.46 | 37.28,34.81 37.03,34.92 36,34.92 arc22 35.87,34.95 35.71,34.93 arc-10 35.54,34.92 35.39,34.95 arc-45 35.3,35.14 35.21,35.27 arc45 34.79,35.46 34.63,35.46 | 37.28,34.81 37.29,34.8
  Top 0.305: 4.37,38.1 USB1.3 5.49,38.1 7.21,37.39 7.92,37.39 Z1.1
D-
  Top 0.254: 7.92,39.01 8.39,39.01 arc-46 8.8,38.62 8.97,38.33 arc46 10.3,37.69 arc-45 13.96,36.33 15.78,34.51 arc45 16.73,33.98 20.05,33.98 arc45 20.26,34.03 arc-45 20.51,34.06 26.37,34.06 arc45 27.02,34.28 28.55,35.81 arc-45 28.99,35.98 29.6,35.98 arc38 29.99,36.11 30.09,36.19 arc-38 30.48,36.3 35.11,36.3 arc-54 35.6,36.06 arc54 36.15,35.83 36.94,35.83 | 7.72,39.01 Z2.1 | U1.38 38.88,34.28 arc45 39.06,34.33 39.28,34.6 arc45 39.32,34.77 39.32,34.87 arc45 39.07,35.35 38.84,35.59 arc45 38.25,35.81 36.98,35.81 R5.1 | USB1.2 4.45,38.75 arc45 4.47,38.76 | R5.1 36.94,35.83 | 36.94,35.83 36.98,35.76 R5.1
  Top 0.305: 4.22,38.76 4.47,38.76 6.04,38.76 7.21,39.01 7.92,39.01 Z2.1 7.91,39.01
DAC0(CANRX1)  (via drill 0.41)
  Top 0.203: v46.02,11.28 45.52,11.28 44.6,12.19 42.67,12.19 41.66,13.21 41.66,15.04 U1.76 | v46.94,8.23 47.85,8.23 48.56,8.94 50.8,8.94 51.21,8.53 59.84,8.53 62.99,11.68 67.87,11.68 73.56,5.99 76.61,5.99 78.13,4.47 80.06,4.47 80.26,4.27 82.09,4.27 ADCH.5 83.72,2.64
  Bottom 0.203: v46.02,11.28 46.74,10.57 46.74,8.64 v46.94,8.23
DAC1  (via drill 0.41)
  Top 0.203: U1.77 42.15,13.33 42.88,12.6 45.41,12.6 v45.72,12.29 | v46.02,8.84 46.13,8.84 46.43,9.14 48.06,9.14 48.26,9.35 51.1,9.35 51.51,8.94 59.64,8.94 62.79,12.09 68.07,12.09 73.76,6.4 77.01,6.4 78.54,4.88 84.02,4.88 ADCH.6
  Bottom 0.203: v45.72,12.29 45.31,11.89 45.31,9.55 v46.02,8.84
DTR
  Top 0.254: IC6.13 18.44,16.24 17.6,15.4 17.6,15.2 16.8,14.4 16.8,12.5 16.3,12 R18.1
EN
  Top 0.406: IC2.4 83.28,12.6 84.33,12.6 84.88,13.15 85.14,13.15 R10.2
ERASE_CMD  (via drill 0.41)
  Top 0.203: T3.3 28.45,15.95 v28.25,15.75
  Top 0.254: IC6.23 21.88,20.76 22.25,21.13 23.27,21.13 23.57,21.44 23.57,22.35 v23.67,22.45
  Top 0.305: R99.1 28.35,16.64 T3.3
  Bottom 0.254: v23.67,22.45 23.67,18.9 24.69,17.88 24.69,16.87 25.6,15.95 28.04,15.95 v28.25,15.75
ERASE_S  (via drill 0.41)
  Top 0.203: v42.57,18.09 42.37,17.88 41.05,17.88 39.83,16.66 36.07,16.66 35.76,16.97 34.34,16.97 33.63,16.26 32.92,16.26 32.72,16.46 30.96,16.46 T3.1 | v45.62,27.74 46.33,27.03 47.55,27.03 47.95,27.43 54.36,27.43 54.56,27.23 57.91,27.23 58.47,27.79 U1.130 60.5,27.79 60.86,28.14 60.86,31.19 60.66,31.39 60.66,32.31 61.06,32.72 61.37,32.72 61.77,33.12 61.77,34.75 62.69,35.66 62.69,36.88 64.62,38.81 67.56,38.81 67.97,39.22 70,39.22 ERASE.2
  Bottom 0.203: v42.57,18.09 42.67,18.09 42.88,17.88 43.59,17.88 44.09,18.39 44.09,18.8 45.41,20.12 45.41,22.55 45.21,22.76 45.21,27.33 v45.62,27.74
FB
  Top 0.61: R12.2 79.43,11.89 R11.1 80.29,11.91 IC2.3
GATE_CMD
  Top 0.203: 17.07,27.61 IC1.7
  Top 0.254: 17.07,27.61 16.43,27.61 16.15,27.33 13.61,27.33 13.41,27.13 13.41,26.42 T1.3
GND  (via drill 0.41, 0.61)
  Top 0.203: 41.66,36.98 U1.33 | 10.36,51.61 RESET.2 | U1.126 59.74,25.79 59.74,25.78 | 57.1,16.97 v57.3,16.97 | R2.1 20.05,42.61 19.61,42.16 19.61,39.93 19.61,39.94 RN1.2
  Top 0.254: IC6.28 18.44,19.51 | C36.2 14.22,20.26 IC6.3 17.54,20.26 17.68,20.12 17.68,20.02 IC6.33 | 56.65,14.58 56.65,13.97 56.79,13.82 | v57.3,16.97 56.64,16.31 56.64,14.58 56.65,14.58 | 56.65,15.19 56.65,14.58 | 65.39,51.04 65.53,50.9 65.94,50.9 66.04,50.8 66.04,49.38 65.6,48.93 | 4.57,35.76 4.57,35.78 USB1.S2 | U1.46 38.92,30.29 39.12,30.48 39.12,31.29
  Top 0.279: 39.12,26.52 38.88,26.29 U1.54 37.05,26.29 36.98,26.21 | U1.33 41.65,38.2 41.64,38.71 | 41.76,38.91 41.64,38.71 | 41.64,38.71 41.64,34.95 | 39.62,31.29 39.12,31.29 U1.44 36.79,31.29 36.78,31.29 | 52.02,38.81 52.15,38.69 U1.12 52.15,35.99 52.02,35.87 | U1.74 40.65,15.13 | 60.8,26.25 60.76,26.21 60.76,26.04 60.5,25.78 59.74,25.78 59.54,25.78 | U1.106 56.65,15.19 | U1.58 39.42,24.29 39.62,24.08 41.1,24.08
  Top 0.305: C31.1 20.09,30.5 v20.22,30.48 | IC1.4 21.37,29.39 v21.74,29.77 22.85,30.88 RN4.2 | RN4.1 23.35,31.68 23.16,31.5 23.16,30.99 23.27,30.89 RN4.2 | RN4.2 RN4.7 25.81,30.88 26.01,30.68 27.13,30.68 v27.94,31.5 28.41,31.03 C24.2 | RN4.5 25.32,29.28 25.3,29.26 25.3,28.25 v25.09,28.04 26.28,28.04 Q2.2 | C23.2 28.41,28.51 v28.96,29.06 | Y1.2 36.54,39.94 Y1.4 | C22.2 33.69,41.9 33.43,42.16 33.43,43.64 DEBUG.1 | IC6.28 18.44,24.2 C30.1 | C38.2 20.36,25.44 v20.62,25.4 | 40.65,15.13 40.65,14.23 40.23,13.82 38.81,13.82 v38.41,14.22 | C28.2 1.73,33.77 | v34.95,24.18 34.95,24.28 34.2,25.03 34.2,25.36 34.24,25.4 | C15.1 34.2,25.67 34.75,26.21 35.56,26.21 | 41.1,24.08 41.6,23.57 v41.99,23.47
  Top 0.356: J3.S3 4.09,26.19 4.06,26.21
  Top 0.406: J3.S1 J3.S5 J3.S6 J3.S2 2.36,18.92 3.15,19.71 4.06,19.71 J3.S4 | J3.S4 Z4.1 6.1,19.41 v6.1,18.19 | v82.09,11.79 82.09,13.11 81.69,13.51 IC2.2 79.63,13.51 R11.2 | J3.P5 J3.S4 | C10.1 38.14,14.49 v38.41,14.22 | RN2.5 18.49,35.15 | 4.37,35.87 arc90 4.55,36.07 4.55,36.78 | 4.47,40.95 4.88,40.95 4.88,42.47
  Top 0.508: C1.- 38.2,9.88 | L.C ON.C 8.98,27.37 v7.82,26.01 | 38.34,14.29 v38.41,14.22
  Top 0.61: 4.57,41.66 4.47,41.66 4.47,40.95
  Top 0.813: C27.- 17.68,46.63 v18.8,47.75 | 73.05,34.75 C29.- 72.82,35.33 72.95,35.26 | v74.68,34.04 v75.84,34.04 78.23,34.04 78.23,34.14 78.26,34.24 IC4.1 | v84.53,17.07 84.56,16.99 D4.P$2 84.68,18.47 C41.- v86.67,20.32 | 13.64,46.81 11.91,46.81 v11.89,46.84 | 4.57,41.66 4.57,40.41 3.15,40.41 | 4.57,34.44 4.57,35.76 | 4.57,35.87 4.57,35.76 | 4.57,35.76 3.15,35.79 4.27,35.79 arc90 4.37,35.87
  Top 1.016: C27.- C35.- 13.64,46.81 | USB1.S2 arc90 4.57,35.77 | USB1.S1 arc-90 4.57,40.43 4.57,40.41 | 4.57,40.41 4.57,40.34 4.67,40.34 arc-90 4.57,40.41
  other vias: 63.2,39.42 49.99,34.04 69.09,38.51 62.38,27.03 38.2,11.38 2.24,4.88 2.24,10.97 8.84,10.77 4.57,33.63 7.82,44.4 99.16,11.61 99.16,19.18 99.16,26.92 99.16,34.44 4.98,42.47 33.32,32.72 71.22,2.44 57.3,34.04 83.97,41.15 6.1,4.88 30.89,32 6.25,51.16 11.28,4.88 7.82,19.81 7.11,16.05 21.13,7.92 25.6,7.92 27.74,36.58 8.23,42.06 29.57,24.08 19.51,20.83 30.99,21.84 31.5,26.52 85.45,20.32 87.78,20.32 62.89,23.88 78.94,17.17 70.51,18.49 66.14,50.8 62.23,49.58 80.92,24.28 14.94,14.02 12.19,38.71 47.98,23.57 22.61,51.71 87.68,48.46 16.87,18.19 22.15,32 71.32,17.68 71.32,19.3 59.69,1.52 29.21,3.61 43.59,50.8 67.67,18.69 65.02,18.69 40.64,31.9 75.95,37.49 77.47,52.12 71.02,26.72 92.76,21.54 87.63,3.56 69.49,6.71 37.8,45.01 57.71,13.41
  pour Top (isolate 0.305, rank 2): 102.11,53.85 102.11,-0.51 -1.02,-0.51 -1.02,52.83 arc-89 0,53.85
  pour Bottom (isolate 0.305, rank 2): -0.51,54.86 103.12,54.86 103.12,-1.52 -1.52,-1.52 -1.52,53.34 arc-90
JTAG_RESET
  Top 0.203: RN1.4 21.15,41.53 21.64,41.05 JTAG.10 | JTAG.10 22.55,41.05 22.55,41.07 | R1.1 22.55,42.47 22.55,41.07 | 22.55,41.07 JTAG.10
JTAG_TCK  (via drill 0.41)
  Top 0.203: RN2.7 18.59,36.73 19.81,36.73 v20.32,37.24 | U1.28 44.15,35.41 v43.89,35.15 | v44.4,46.13 44.3,46.02 42.37,46.02 42.16,46.23 37.39,46.23 37.19,46.43 v30.68,46.43 30.48,46.23 22.15,46.23 21.34,45.41 v20.32,45.41
  Bottom 0.203: JTAG.4 v20.32,37.24 20.32,38.51 20.12,38.71 20.12,44.7 20.32,44.91 v20.32,45.41 | v43.89,35.15 44.09,35.36 44.09,38.71 44.4,39.01 v44.4,46.13
  Bottom 0.254: DEBUG.2 30.68,43.54 v30.68,46.43
JTAG_TDI  (via drill 0.41)
  Top 0.203: v22.05,48.16 22.35,48.16 22.66,47.85 26.82,47.85 27.53,48.56 28.75,48.56 28.96,48.36 37.8,48.36 38.3,48.87 43.18,48.87 v43.28,48.77 | U1.29 43.64,37.67 43.69,37.72 v43.69,39.32
  Top 0.254: RN1.3 20.83,40.73 21.74,39.83 22.48,39.83 JTAG.8
  Bottom 0.203: v43.69,39.32 43.38,39.62 43.38,46.02 43.69,46.33 43.69,48.26 v43.28,48.77 | v22.05,48.16 22.05,45.21 21.54,44.7 21.54,44.3 21.13,43.89 21.13,40.23 21.54,39.83 22.55,39.83 22.53,39.8 JTAG.8
JTAG_TDO  (via drill 0.41)
  Top 0.203: v42.98,46.74 42.88,46.63 37.69,46.63 37.19,47.14 29.16,47.14 28.65,46.63 21.84,46.63 21.54,46.33 v21.03,46.33 | U1.30 43.13,36.8 43.13,36.58 43.18,36.58 v43.18,34.34
  Bottom 0.203: v21.03,46.33 21.03,44.7 20.62,44.3 20.62,39.55 21.67,38.51 JTAG.6 | v42.98,46.74 42.98,38.96 43.18,38.76 v43.18,34.34
JTAG_TMS  (via drill 0.41)
  Top 0.203: v19.51,35.92 18.59,35.92 RN2.6 | v42.47,38.41 42.65,38.23 42.65,37.01 U1.31 | v41.96,47.35 41.66,47.04 38,47.04 37.49,47.55 28.25,47.55 v28.14,47.45 27.84,47.45 27.43,47.04 20.42,47.04 19.61,46.23 v19.51,46.23
  Bottom 0.203: v41.96,47.35 41.96,38.91 v42.47,38.41 | v19.51,46.23 v19.51,35.92 22.5,35.92 JTAG.2 | JTAG.2 22.55,35.97 22.55,35.94 JTAG.2 | DEBUG.3 28.14,43.54 v28.14,47.45
L13
  Top 0.203: 21.34,26.98 IC1.1 | RN3.6 14.79,30.54 14.94,30.48 16.05,30.48 16.87,31.29 20.42,31.29 20.93,30.79 20.93,29.97 20.32,29.36 20.32,27.8 20.5,27.61
  Top 0.305: 21.34,26.98 20.32,26.98 20.32,27.43 20.5,27.61 IC1.2
MASTER-RESET  (via drill 0.41)
  Top 0.203: 9.14,46.53 RESET.4 10.46,46.56 10.46,47.45 10.77,47.75 17.58,47.75 18.8,48.97 22.35,48.97 23.06,48.26 26.52,48.26 27.23,48.97 28.96,48.97 29.16,48.77 30.38,48.77 30.68,49.07 v30.89,49.07 | U1.47 39.23,29.79 40.03,30.58 v40.34,30.58 | SPI.5 63.6,25.4 | v62.08,6.1 59.23,6.1 59.03,6.3 57.1,6.3 56.08,7.32 51,7.32 50.7,7.01 49.38,7.01 48.87,7.52 48.16,7.52 46.43,5.79 45.06,5.79 44.86,5.99 34.44,5.99 v34.24,5.79 | v25.45,19 23.88,19 23.41,19.47 R23.2 | R1.2 25.41,43.73 | v30.79,17.68 32.11,18.59 33.53,18.59 33.63,18.49 v34.04,18.49
  Top 0.254: v31.09,41.45 30.48,42.06 26.72,42.06 25.65,43.13 DEBUG.4 25.41,43.73
  Top 0.305: 2.54,46.52 3.96,46.52 3.96,46.53 9.14,46.53 10.06,46.53 | 2.54,46.52 RESET.3 | RESET.4 10.42,46.63 10.06,46.63 10.06,46.53 | 10.06,46.53 10.46,46.53 | C20.1 2.68,46.38 2.54,46.52
  Bottom 0.203: v30.89,49.07 30.89,48.36 31.7,47.55 36.98,47.55 38.61,45.92 38.61,44.7 39.62,43.69 39.62,38.41 40.54,37.49 40.54,34.14 41.66,33.02 41.66,31.39 40.84,30.58 v40.34,30.58 | SPI.5 63.6,25.4 64.36,24.64 64.36,24.43 66.34,22.45 66.34,14.33 61.67,9.65 61.67,6.71 62.08,6.3 v62.08,6.1 | POWER.3 33.02,4.57 v34.24,5.79 34.04,5.99 v34.04,18.49 34.04,19.41 32.72,20.73 32.72,23.98 31.29,25.4 31.29,25.7 30.79,26.21 30.58,26.21 30.28,26.52 30.28,31.5 29.26,32.51 29.26,39.62 v31.09,41.45 | v30.79,17.68 30.48,17.58 30.38,17.58 29.97,17.98 29.97,19 29.16,19.81 26.26,19.81 v25.45,19
  Bottom 0.254: 31.7,47.55 31.7,44.91 32,44.6 32,42.37 v31.09,41.45
MISO  (via drill 0.41)
  Top 0.203: U1.108 57.71,16.15 58.32,16.76 60.96,16.76 62.69,18.49 64.01,18.49 64.72,17.78 68.89,17.78 v69.09,17.98
  Bottom 0.203: 63.6,30.48 SPI.1 64.01,30.48 65.23,29.26 67.87,29.26 69.19,27.94 69.19,27.23 69.49,26.92 69.49,25.91 69.9,25.5 69.9,22.15 69.09,21.34 v69.09,17.98
MISO2  (via drill 0.41)
  Top 0.203: IC6.17 20.64,16.96 v20.73,16.87
  Bottom 0.203: v20.73,16.87 20.22,16.87 19.71,16.36 19.71,15.34 20.02,15.04 21.34,15.04 22.86,13.51 24.64,13.51 ICSP1.1
MOSI  (via drill 0.41)
  Top 0.203: U1.109 59.74,17.27 60.76,17.27 62.69,19.2 63.5,19.2 63.8,19.51 66.55,19.51 68.28,21.23 v70.41,21.23 | 66.14,27.94 SPI.4 66.17,27.96 66.14,27.94
  Top 0.305: 66.14,27.94 67.26,27.94 67.67,27.53 v70,27.53
  Bottom 0.203: v70,27.53 70,26.21 70.41,25.81 v70.41,21.23
MOSI2  (via drill 0.41)
  Top 0.254: IC6.16 19.94,16.54 v20.73,15.75
  Bottom 0.203: v20.73,15.75 22.15,15.75 23.16,14.73 ICSP1.4
N$1
  Top 0.203: IC6.26 19.44,22.48 19.81,22.86 20.12,22.86 20.42,23.16 20.56,23.16 R21.1
N$2
  Top 0.254: L.A 12.56,30.54 RN3.3
N$3
  Top 0.254: RN3.4 13.22,29.31 ON.A
N$4
  Top 0.254: 3.21,16.91 3.25,16.87 RX1.A 2.03,15.68 R15.2
N$5
  Top 0.203: U1.51 35.76,27.79 R8.2
N$6  (via drill 0.41)
  Top 0.203: 25.4,31.7 RN4.8
  Top 0.279: 27.13,25.4 26.82,25.4 26.42,25.81 26.42,25.8 Q2.1
  Top 0.305: v26.42,31.5 26.21,31.7 25.4,31.7 | 27.13,25.4 R3.2 28.65,25.4
  Top 0.356: R3.2 28.41,26.15 v27.84,26.72
  Bottom 0.203: v27.84,26.72 26.72,27.84 26.72,31.19 v26.42,31.5
N$7
  Top 0.203: U1.53 38,26.82 34.65,26.82 33.53,25.76 33.53,25.7 33.22,25.4 R4.1
N$10
  Top 1.016: L6.1 15.79,8.86 D5.P$2
N$11
  Top 0.203: U1.43 39.3,31.79 40.34,32.82 40.34,35.31 38.96,36.68 36.74,36.68 | 36.73,36.68 36.74,36.68 | 36.74,36.68 36.73,36.68 | 36.73,36.68 36.74,36.68 | 36.74,36.68 R5.2 | 36.73,36.68 36.74,36.68 | 36.74,36.68 36.73,36.68 | 36.73,36.68 36.74,36.68 | 36.74,36.68 36.73,36.68 | 36.73,36.68 36.74,36.68
N$12
  Top 0.203: U1.42 38,32.31 36.58,32.31 36.17,31.9 33.02,31.9 32.51,32.41 32.51,33.83 33.24,34.56 R6.2
N$14
  Top 0.254: R14.2 3.35,13.45 TX1.A
N$54
  Top 0.254: RN3.1 11.97,33.36 RX.A
N$55
  Top 0.254: RN3.2 11.89,31.34 arc90 TX.A
PIN22  (via drill 0.41)
  Top 0.203: v60.25,37.39 60.05,37.19 57.61,37.19 U1.1 | v66.04,46.23 66.34,45.92 68.07,45.92 68.28,45.72 73.15,45.72 73.76,46.33 77.42,46.33 77.83,46.74 79.86,46.74 80.37,47.24 91.75,47.24 92.76,48.26 XIO.3
  Bottom 0.203: v60.25,37.39 60.76,37.39 61.77,38.41 61.77,40.03 60.86,40.95 60.86,46.33 61.06,46.53 65.73,46.53 v66.04,46.23
PIN23  (via drill 0.41)
  Top 0.203: v59.64,39.42 58.42,39.42 58.12,39.12 55.8,39.12 54.66,37.97 54.66,36.98 U1.7 | v69.6,47.35 70.81,46.13 72.95,46.13 73.56,46.74 77.22,46.74 77.62,47.14 79.65,47.14 80.16,47.65 91.34,47.65 93.27,49.58 95.2,49.58 XIO.4
  Bottom 0.203: v59.64,39.42 59.64,46.94 60.45,47.75 69.19,47.75 v69.6,47.35
PIN24  (via drill 0.41)
  Top 0.203: XIO.5 92.46,45.72 91.34,44.6 87.17,44.6 86.56,45.21 81.38,45.21 80.87,44.7 78.84,44.7 78.44,44.3 74.78,44.3 74.17,43.69 67.26,43.69 67.06,43.89 64.92,43.89 63.3,45.52 60.15,45.52 59.33,44.7 54.56,44.7 v54.25,44.4 | U1.8 54.15,37.89 54.25,38 v54.25,38.91
  Bottom 0.203: v54.25,44.4 v54.25,38.91
PIN25  (via drill 0.41)
  Top 0.203: v51.36,38.2 51.64,37.92 51.64,36.96 U1.13 | v51.51,46.63 51.82,46.33 58.52,46.33 59.33,47.14 64.11,47.14 65.73,45.52 67.87,45.52 68.07,45.31 73.36,45.31 73.97,45.92 77.62,45.92 78.03,46.33 80.06,46.33 80.57,46.84 92.15,46.84 92.25,46.94 95.3,46.94 XIO.6
  Bottom 0.203: v51.51,46.63 52.73,45.52 52.73,39.83 51.71,38.81 51.71,38.56 v51.36,38.2
PIN26  (via drill 0.41)
  Top 0.203: XIO.7 92.56,43.18 91.75,43.79 86.77,43.79 86.16,44.4 81.79,44.4 81.28,43.89 79.25,43.89 78.84,43.48 75.18,43.48 74.57,42.88 66.85,42.88 66.65,43.08 64.52,43.08 62.89,44.7 60.55,44.7 59.74,43.89 55.37,43.89 54.76,43.28 53.65,43.28 52.93,43.99 v52.02,43.99 | U1.14 51.15,35.91 v50.39,35.15
  Bottom 0.203: v52.02,43.99 52.02,39.9 50.6,38.48 50.6,35.36 v50.39,35.15
PIN27  (via drill 0.41)
  Top 0.203: XIO.8 95.2,44.5 92.05,44.5 91.75,44.2 86.97,44.2 86.36,44.81 81.58,44.81 81.08,44.3 79.05,44.3 78.64,43.89 74.98,43.89 74.37,43.28 67.06,43.28 66.85,43.48 64.72,43.48 63.09,45.11 60.35,45.11 59.54,44.3 55.17,44.3 54.56,43.69 53.85,43.69 52.83,44.7 51.31,44.7 v51,44.4 | v50.49,39.42 50.49,38.99 50.65,38.84 U1.15 50.65,36.83
  Bottom 0.203: v51,44.4 51,39.93 v50.49,39.42
PIN28  (via drill 0.41)
  Top 0.203: U1.16 50.14,36.78 50.14,37.85 50.19,37.9 50.19,38.6 50.2,38.7 49.78,39.12 v49.78,40.23 | v49.99,43.18 51,43.18 51.31,42.88 52.83,42.88 53.24,42.47 55.17,42.47 55.78,43.08 60.15,43.08 60.96,43.89 62.48,43.89 64.11,42.27 66.24,42.27 66.45,42.06 74.98,42.06 75.59,42.67 79.25,42.67 79.65,43.08 81.69,43.08 82.19,43.59 85.75,43.59 86.36,42.98 90.93,42.98 92.46,41.66 92.56,41.66 92.96,41.25 93.37,41.25 XIO.9
  Bottom 0.203: v49.78,40.23 49.78,42.98 v49.99,43.18
PIN29  (via drill 0.41)
  Top 0.203: XIO.10 95.3,41.86 93.07,41.86 91.34,43.38 86.56,43.38 85.95,43.99 81.99,43.99 81.48,43.48 79.45,43.48 79.05,43.08 75.39,43.08 74.78,42.47 66.65,42.47 66.45,42.67 64.31,42.67 62.69,44.3 60.76,44.3 59.94,43.48 55.58,43.48 54.97,42.88 53.44,42.88 53.03,43.28 51.61,43.28 51.21,43.69 50.6,43.69 50.09,44.2 48.16,44.2 47.55,44.81 47.55,45.21 v47.14,45.62 | U1.19 48.65,37.88 48.77,38 48.77,38.91 48.16,39.52 v46.74,39.52
  Bottom 0.203: v46.74,39.52 46.74,45.21 v47.14,45.62
PIN30  (via drill 0.41)
  Top 0.203: 47.14,36.78 U1.22 47.15,36.78 47.14,36.78 | 47.14,36.78 47.14,37.69 46.94,37.9 46.94,38.2 v46.63,38.51 | v47.65,47.85 47.85,47.85 49.78,45.92 58.73,45.92 59.54,46.74 63.91,46.74 65.53,45.11 67.67,45.11 67.87,44.91 73.56,44.91 74.17,45.52 77.83,45.52 78.23,45.92 80.26,45.92 80.77,46.43 89.2,46.43 v89.61,46.02
  Bottom 0.203: XIO.11 91.08,38.1 89.51,39.67 89.51,44.7 89.61,44.81 v89.61,46.02 | v46.63,38.51 46.02,39.12 46.02,44.81 46.33,45.11 46.33,45.92 47.65,47.24 v47.65,47.85
PIN31  (via drill 0.41)
  Top 0.203: v45.21,38.2 45.14,38.12 45.14,37.11 U1.26 | v45.82,47.14 47.95,47.14 49.58,45.52 58.93,45.52 59.74,46.33 63.7,46.33 65.33,44.7 67.46,44.7 67.67,44.5 73.76,44.5 74.37,45.11 78.03,45.11 78.44,45.52 80.47,45.52 80.97,46.02 87.99,46.02 v88.7,45.31 | v89,38.61 92.56,38.61 93.37,39.42 95.2,39.42 XIO.12
  Bottom 0.203: v45.82,47.14 45.82,46.74 45.52,46.43 45.52,45.52 45.21,45.21 v45.21,38.2 | v89,38.61 89,42.57 88.7,42.88 v88.7,45.31
PIN32  (via drill 0.41)
  Top 0.203: U1.32 42.15,35.48 v42.47,35.15 | v87.58,36.17 88.19,35.56 XIO.13 94.08,35.56 | v44.4,47.14 45.11,46.43 46.23,46.43 46.53,46.74 47.75,46.74 49.38,45.11 59.13,45.11 59.94,45.92 63.5,45.92 65.13,44.3 67.26,44.3 67.46,44.09 73.97,44.09 74.57,44.7 78.23,44.7 78.64,45.11 80.67,45.11 81.18,45.62 87.27,45.62 v87.58,45.31
  Bottom 0.203: v42.47,35.15 42.47,37.39 41.25,38.61 41.25,47.75 42.16,48.67 42.16,48.97 42.67,49.48 43.79,49.48 44.4,48.77 v44.4,47.14 | v87.58,45.31 v87.58,36.17
PIN33  (via drill 0.41)
  Top 0.203: v56.69,28.35 56.39,28.04 54.97,28.04 54.76,28.25 49.48,28.25 49.28,28.45 43.59,28.45 42.88,27.74 40.34,27.74 39.73,27.13 39.73,26.42 39.12,25.81 38.2,25.81 U1.55 | v88.29,42.27 87.99,42.57 86.16,42.57 85.55,43.18 82.4,43.18 81.89,42.67 79.86,42.67 79.45,42.27 75.79,42.27 75.18,41.66 66.24,41.66 66.04,41.86 63.91,41.86 62.28,43.48 61.16,43.48 60.35,42.67 57.71,42.67 v57.4,42.37 | v88.29,37.8 89.31,36.78 95.3,36.78 XIO.14
  Bottom 0.203: v88.29,37.8 v88.29,42.27 | v56.69,28.35 57.1,28.75 58.62,28.75 60.05,30.18 60.05,34.04 57.51,36.58 57.51,39.83 58.12,40.44 58.12,41.66 v57.4,42.37
PIN34  (via drill 0.41)
  Top 0.203: v56.79,23.98 56.59,23.98 55.88,23.27 52.93,23.27 52.02,22.35 42.06,22.35 40.79,23.62 39.37,23.62 39.22,23.77 38.2,23.77 U1.59 | XIO.15 92.96,33.02 90.73,30.79 90.22,30.79 88.29,28.85 80.26,28.85 79.96,28.55 74.37,28.55 73.36,29.57 69.8,29.57 69.6,29.36 v68.89,29.36
  Bottom 0.203: v68.89,29.36 66.34,31.9 62.99,31.9 62.18,31.09 62.18,29.87 58.73,26.42 57.51,26.42 56.79,25.7 v56.79,23.98
PIN35  (via drill 0.41)
  Top 0.203: U1.60 39.1,23.29 39.22,23.16 40.64,23.16 41.86,21.95 52.22,21.95 53.14,22.86 56.08,22.86 56.49,23.27 57.4,23.27 58.01,23.88 v58.12,23.88 | XIO.16 95.2,31.7 92.86,31.7 92.66,31.5 92.66,29.77 91.64,28.75 89.51,28.75 88.8,28.04 80.67,28.04 80.37,27.74 73.46,27.74 70.92,25.2 68.07,25.2 v67.87,25.4
  Bottom 0.203: v58.12,23.88 60.35,23.88 63.09,26.62 64.41,26.62 64.87,26.16 64.87,24.79 65.4,24.25 65.87,23.77 66.34,23.77 67.87,25.3 v67.87,25.4
PIN36
  Top 0.203: U1.116 59.7,20.77 59.79,20.78 60.5,20.78 61.16,21.44 61.77,21.44 63.3,22.96 65.63,22.96 67.36,24.69 71.02,24.69 73.66,27.33 80.67,27.33 80.87,27.53 89,27.53 89.81,28.35 91.85,28.35 XIO.17
PIN37  (via drill 0.41)
  Top 0.203: v68.89,32.72 62.99,32.72 62.89,32.61 62.08,32.61 v61.37,31.9 | U1.63 38.2,21.74 39.42,21.74 39.62,21.54 52.43,21.54 53.34,22.45 56.69,22.45 v56.79,22.55 | v91.34,29.57 89.71,29.57 88.59,28.45 80.47,28.45 80.16,28.14 v71.02,28.14
  Bottom 0.203: v56.79,22.55 55.58,22.55 54.76,23.37 54.76,24.99 57,27.23 58.32,27.23 61.37,30.28 v61.37,31.9 | v91.34,29.57 91.64,29.26 95.3,29.26 XIO.18 | v71.02,28.14 71.02,30.68 v68.89,32.72
PIN38  (via drill 0.41)
  Top 0.203: U1.64 39.27,21.29 39.42,21.13 52.63,21.13 53.54,22.05 56.29,22.05 56.49,21.84 57.1,21.84 v58.12,22.86 | v64.31,22.25 65.53,22.25 67.56,24.28 71.22,24.28 73.86,26.92 80.97,26.92 81.18,27.13 89.31,27.13 90.12,27.94 XIO.19
  Bottom 0.203: v58.12,22.86 58.42,22.55 64.01,22.55 v64.31,22.25
PIN39  (via drill 0.41)
  Top 0.203: U1.65 39.16,20.79 39.22,20.73 52.83,20.73 53.75,21.64 56.08,21.64 56.59,21.13 v57.1,21.13 | v62.48,21.13 65.73,21.13 68.07,23.47 71.63,23.47 74.27,26.11 81.58,26.11 81.79,26.31 89.92,26.31 90.22,26.62 v91.34,26.62
  Bottom 0.203: v57.1,21.13 57.2,21.13 57.3,21.03 58.73,21.03 58.83,21.13 60.55,21.13 60.76,21.34 62.28,21.34 v62.48,21.13 | v91.34,26.62 95.2,26.62 XIO.20
PIN40  (via drill 0.41)
  Top 0.203: U1.66 39.18,20.29 39.22,20.32 53.03,20.32 53.95,21.23 55.88,21.23 56.69,20.42 57.4,20.42 58.12,21.13 v58.12,21.74 | v63.25,21.84 63.7,21.84 64.01,21.54 65.43,21.54 67.77,23.88 71.42,23.88 74.07,26.52 81.28,26.52 81.48,26.72 89.61,26.72 90.42,27.53 91.85,27.53 XIO.21
  Bottom 0.203: v58.12,21.74 60.35,21.74 60.45,21.84 v63.25,21.84
PIN41  (via drill 0.41)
